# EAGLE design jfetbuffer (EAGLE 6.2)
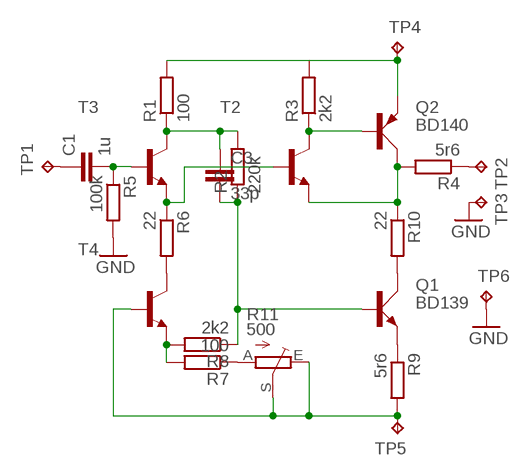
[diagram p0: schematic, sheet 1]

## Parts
C1  1u  C5/7.2  [C5B7.2]
C3  33p  C5/2.5  [C5B2.5]
Q1  BD139  [TO126AV]
Q2  BD140  [TO126AV]
R1  100  R-EU_0207/10  [0207/10]
R2  220k  R-EU_0207/10  [0207/10]
R3  2k2  R-EU_0207/10  [0207/10]
R4  5r6  R-EU_0207/10  [0207/10]
R5  100k  R-EU_0207/10  [0207/10]
R6  22  R-EU_0207/10  [0207/10]
R7  100  R-EU_0207/10  [0207/10]
R8  2k2  R-EU_0207/10  [0207/10]
R9  5r6  R-EU_0207/10  [0207/10]
R10  22  R-EU_0207/10  [0207/10]
R11  500  TRIM_EU-B64Y  [B64Y]
T2  BC239-NPN-TO92-CBE  [TO92-CBE]
T3  BC239-NPN-TO92-CBE  [TO92-CBE]
T4  BC239-NPN-TO92-CBE  [TO92-CBE]
TP1  TPPAD1-13Y  [P1-13Y]
TP2  TPPAD1-13Y  [P1-13Y]
TP3  TPPAD1-13Y  [P1-13Y]
TP4  TPPAD1-13Y  [P1-13Y]
TP5  TPPAD1-13Y  [P1-13Y]
TP6  TPPAD1-13Y  [P1-13Y]

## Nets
GND: R5.2 TP3.TP TP6.TP
N$1: Q2.B R3.1 T2.C
N$2: C3.1 R1.1 R2.2 T3.C
N$3: C1.2 R5.1 T3.B
N$4: R6.1 T2.B T3.E
N$5: R6.2 T4.C
N$6: R7.2 R8.2 T4.E
N$7: Q2.C R4.2 R10.1 T2.E
N$8: Q1.E R9.1
N$9: Q1.C R10.2
N$10: C3.2 Q1.B R2.1 R8.1
N$11: R7.1 R11.A
N$12: Q2.E R1.2 R3.2 TP4.TP
N$13: C1.1 TP1.TP
N$14: R4.1 TP2.TP
N$18: R9.2 R11.E R11.S T4.B TP5.TP

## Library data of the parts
C1 C3 = capacitor-wima:C: CAPACITOR
Q1 = transistor-power:BD139: NPN TRANSISTOR
Q2 = transistor-power:BD140: PNP TRANSISTOR
R1-R10 = rcl:R-EU_: RESISTOR, European symbol
R11 = pot:TRIM_EU-: POTENTIOMETER
T2-T4 = transistor:*-NPN-: NPN Transistror BF959 corrected 2008.03.06
TP1-TP6 = testpad:TP: Test pad

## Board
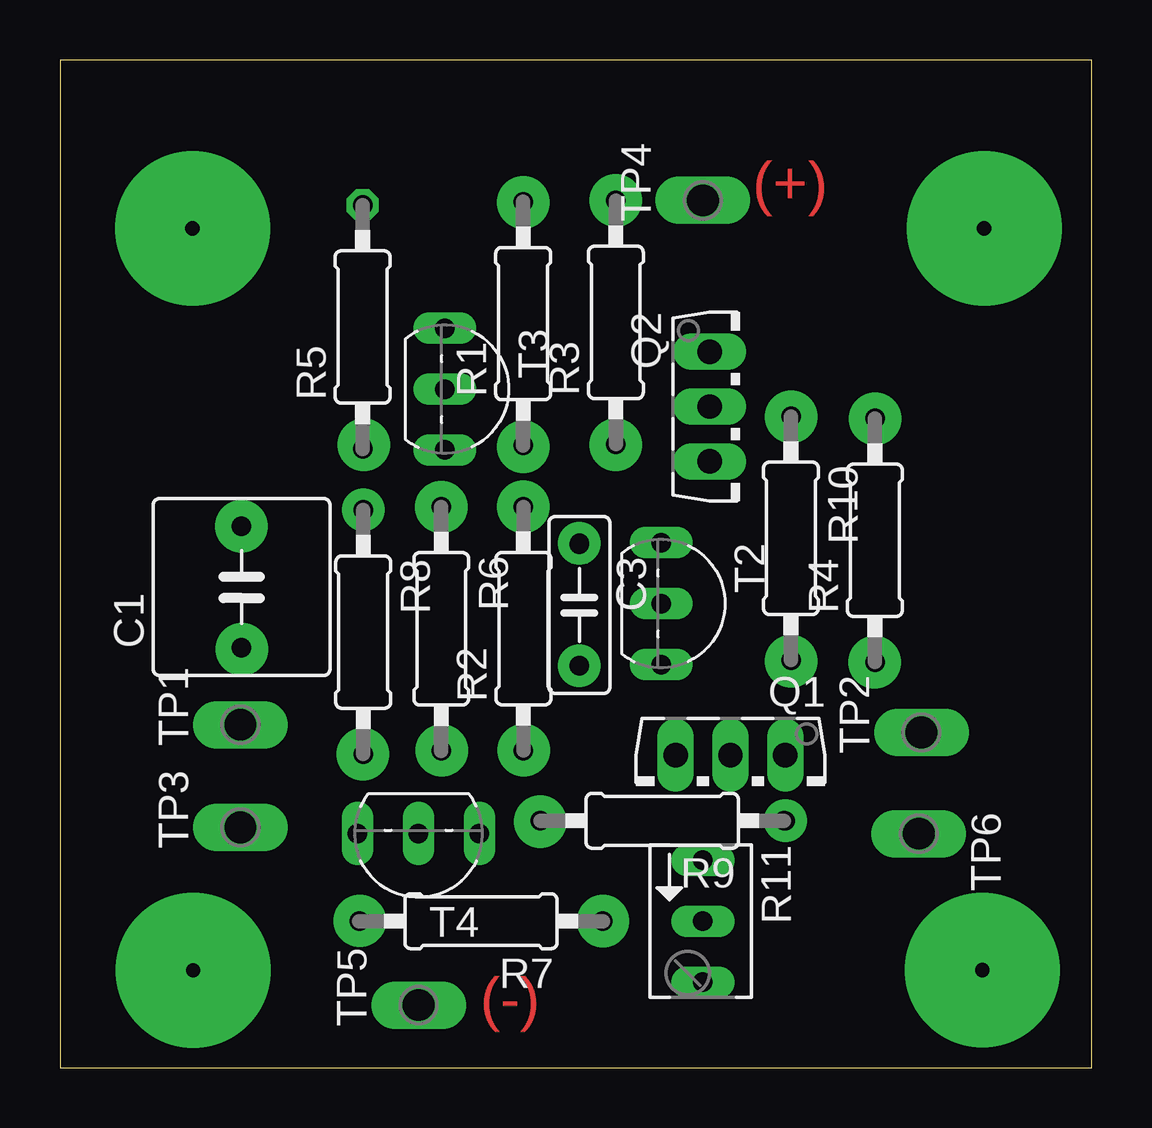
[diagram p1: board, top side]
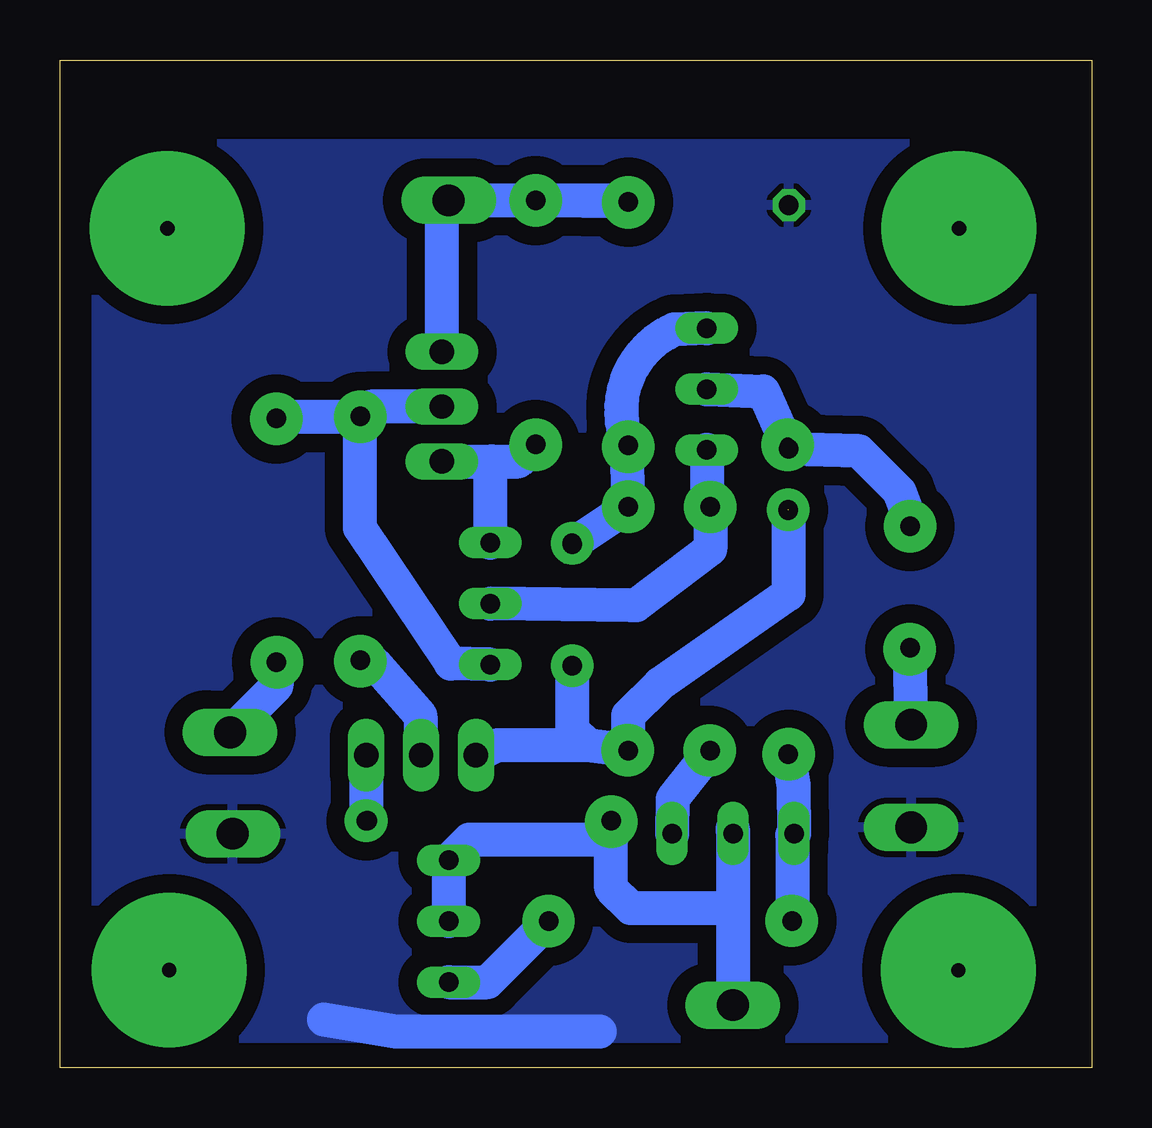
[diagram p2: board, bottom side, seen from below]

Size 43 x 42 mm. Coordinates in mm from the lower left corner, seen from the top.
Outline: 0,0 43,0 43,42 0,42 0,0
Copper layers (1*16): Top 0.035mm / dielectric 1.5mm / Bottom 0.035mm
Design rules: minimum track width 10mil, minimum drill 24mil, track to track 30mil, track to pad 30mil, pad to pad 30mil, via to via 30mil, smd to smd 30mil, copper to edge 40mil, drill to drill 8mil, minimum pad ring 10mil, minimum via ring 8mil, stop-mask expansion 4mil, vias tented up to drill 0mil, thermal gap 10mil

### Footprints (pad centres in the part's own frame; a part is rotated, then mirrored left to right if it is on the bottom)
C5B7.2 = drill 0.813 pad 1.6 octagon: 1 -2.54,0; 2 2.54,0
C5B2.5 = drill 0.813 pad 1.6 octagon: 1 -2.54,0; 2 2.54,0
TO126AV = drill 1.016 long: B 2.286,-1.27; C 0,-1.27; E -2.286,-1.27
0207/10 = drill 0.813 octagon: 1 -5.08,0; 2 5.08,0
B64Y = drill 0.813 long: A 2.54,0; E -2.54,0; S 0,0
TO92-CBE = drill 0.813 long: B 0,0; C -2.54,0; E 2.54,0
P1-13Y = drill 1.321 pad 1.905 long: TP 0,0

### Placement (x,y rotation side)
C1  7.57,20.03 90 top
C3  21.65,19.28 270 top
Q1  27.95,11.75 180 top
Q2  28.35,27.55 270 top
R1  19.31,31.01 90 top
R2  19.32,18.3 90 top
R3  23.17,31.06 90 top
R4  33.97,21.98 90 top
R5  12.62,30.87 90 top
R6  15.89,18.29 270 top
R7  17.55,6.1 180 top
R8  12.64,18.15 270 top
R9  25.11,10.28 180 top
R10  30.47,22.06 270 top
R11  26.8,6.1 270 top
T2  25.06,19.34 270 top
T3  16.04,28.28 270 top
T4  14.94,9.76 180 top
TP1  7.52,14.29 90 top
TP2  35.91,13.97 90 top
TP3  7.52,10.01 90 top
TP4  26.8,36.15 90 top
TP5  14.95,2.6 90 top
TP6  35.8,9.75 270 top

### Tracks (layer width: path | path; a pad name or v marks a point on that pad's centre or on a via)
GND
  Bottom 1.422: 20.5,1.5 29,1.5 32,2
  pour Bottom: 2.5,38.5 41.5,38.5 41.5,1 2.5,1
N$1
  Bottom 1.422: Q2.B 25,25.26 | 25,25.26 23.89,25.26 R3.1 | T2.C 25.06,25.21 25,25.26
N$2
  Bottom 1.422: T3.C 17.39,30.76 arc-90 R1.1 19.34,26.06 R2.2 21.62,21.85 C3.1
N$3
  Bottom 1.422: C1.2 arc-90 7.52,22.72 8,24 9.69,25.69 R5.1 13.68,28.18 T3.B
N$4
  Bottom 1.422: T3.E 16.04,23.72 arc90 R6.1 15.89,21.61 18.97,19.27 19.19,19.27 T2.B
N$5
  Bottom 1.422: R6.2 17.46,11.2 T4.C
N$6
  Bottom 1.422: R8.2 12.42,11.74 T4.E 12.47,9.68 R7.2
N$7
  Bottom 1.422: T2.E 26.7,16.84 30.5,22.5 30.5,27.11 | 30.5,27.11 R10.1 30.06,27.55 Q2.C | 30.5,27.11 33.92,27.11 R4.2
N$8
  Bottom 1.422: Q1.E 30.24,10.34 R9.1
N$9
  Bottom 1.422: R10.2 30.44,16.95 29.9,16.86 27.97,14.66 28,13.07 Q1.C
N$10  (via drill 0.8 pad 1.78)  (1 unrouted)
  Bottom 1.422: R8.1 12.63,19.73 18,16 19.32,14.68 R2.1 21,13.43 | 21,13.43 24.75,13.43 Q1.B | C3.2 21.65,14.08 21,13.43
  other vias: 12.65,23.25
N$11
  Bottom 1.422: R11.A 25.17,3.56 R7.1
N$12
  Bottom 1.422: R3.2 R1.2 19.78,36.15 TP4.TP 27.08,35.87 Q2.E
N$13
  Bottom 1.422: TP1.TP C1.1
N$14
  Bottom 1.422: R4.1 33.97,15.91 TP2.TP
N$16  (via drill 0.6 pad 2.18)
  other vias: 19.31,25.88
N$17  (via drill 0.6 pad 2.18)
  other vias: 30.48,16.95
N$18
  Bottom 1.422: T4.B 14.95,9.96 14.95,6.3 | 14.95,6.3 TP5.TP | 14.95,6.3 15.3,6.65 19.2,6.65 20.03,7.48 R9.2 20.03,9.5 25.94,9.5 R11.E R11.S
N$19  (via drill 0.6 pad 2.18)
  other vias: 12.62,13.05
N$20  (via drill 0.6 pad 2.18)
  other vias: 15.92,13.22
N$21  (via drill 0.6 pad 2.18)
  other vias: 12.49,6.11
N$22  (via drill 0.8 pad 1.78)
  other vias: 30.24,10.28
N$23  (via drill 0.6 pad 2.18)
  other vias: 19.31,23.38
N$24  (via drill 0.6 pad 2.18)
  other vias: 15.9,23.37
N$25  (via drill 0.6 pad 2.18)
  other vias: 23.17,25.97
N$26  (via drill 0.6 pad 2.18)
  other vias: 19.33,13.23
N$27  (via drill 0.6 pad 2.18)
  other vias: 20.02,10.25
N$28  (via drill 0.6 pad 2.18)
  other vias: 30.48,27.12
N$29  (via drill 0.6 pad 2.18)
  other vias: 33.97,16.9
N$32  (via drill 0.6 pad 2.18)
  other vias: 33.98,27.04
N$33  (via drill 0.6 pad 2.18)
  other vias: 23.17,36.14
N$34  (via drill 0.6 pad 2.18)
  other vias: 19.31,36.06
N$35  (via drill 0.6 pad 2.18)
  other vias: 12.66,25.96
N$36  (via drill 0.6 pad 2.18)
  other vias: 7.56,22.56
N$37  (via drill 0.6 pad 2.18)
  other vias: 22.64,6.1
N$38  (via drill 0.6 pad 2.18)
  other vias: 7.58,17.44
N$39  (via drill 0.6 pad 6.45)
  other vias: 38.53,34.98
N$40  (via drill 0.6 pad 6.45)
  other vias: 38.45,4.06
N$41  (via drill 0.6 pad 6.45)
  other vias: 5.55,4.05
N$42  (via drill 0.8 pad 1.78)
  other vias: 21.65,16.75
N$43  (via drill 0.8 pad 1.78)
  other vias: 21.65,21.85
N$44  (via drill 0.6 pad 6.45)
  other vias: 5.53,34.98

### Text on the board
Top: (+) | (-)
